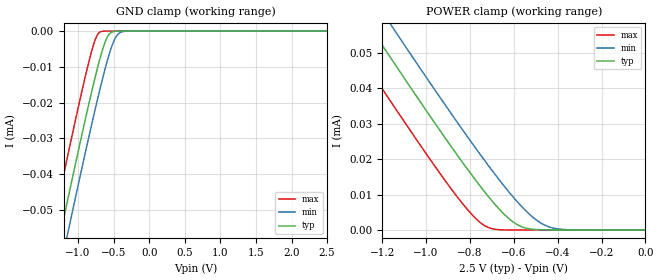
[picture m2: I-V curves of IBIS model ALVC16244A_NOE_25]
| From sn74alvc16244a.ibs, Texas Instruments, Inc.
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[Model]   ALVC16244A_NOE_25
Model_type  Input
Vinl=0.7
Vinh=1.7
| variable   typ   min   max
C_comp   0.77pF   0.49pF   0.91pF
[Temperature Range]   40   100   -40
| Ambient temperature   25   85   -40
[Voltage range]   2.5   2.3   2.7
[GND Clamp]
| ALVC16244A_NOE_25
|   Voltage   I(typ)   I(min)   I(max)
-2.5V     -176.3uA   -185.4uA   -164.4uA
-1.36V    -67.24uA   -76.66uA   -54.98uA
-1.225V   -54.58uA   -64.02uA   -42.29uA
-1.15V    -47.61uA   -57.05uA   -35.31uA
-1.115V   -44.37uA   -53.81uA   -32.07uA
-825mV    -18.36uA   -27.57uA   -6.799uA
-755mV    -12.54uA   -21.51uA   -2.209uA
-695mV    -7.907uA   -16.49uA   -307.2nA
-565mV    -939.8nA   -6.679uA   -650.9pA
-475mV    -50.26nA   -1.907uA   -14.65pA
-380mV    -1.649nA   -181.8nA   -6.292pA
2.5V      4.712pA    817.3pA    4.189pA
[POWER Clamp]
| ALVC16244A_NOE_25
|   Voltage   I(typ)   I(min)   I(max)
-2.5V     176.3uA    185.4uA    164.4uA
-1.4V     71uA       80.42uA    58.76uA
-1.34V    65.35uA    74.78uA    53.09uA
-1.235V   55.51uA    64.95uA    43.22uA
-1.145V   47.14uA    56.59uA    34.84uA
-915mV    26.21uA    35.56uA    14.14uA
-785mV    14.99uA    24.09uA    3.967uA
-710mV    9.02uA     17.73uA    561.4nA
-595mV    1.93uA     8.747uA    2.773nA
-500mV    121nA      2.949uA    33.97pA
-425mV    8.361nA    622.1nA    7.082pA
-31.15fV  4.712pA    6.41pA     4.886pA
